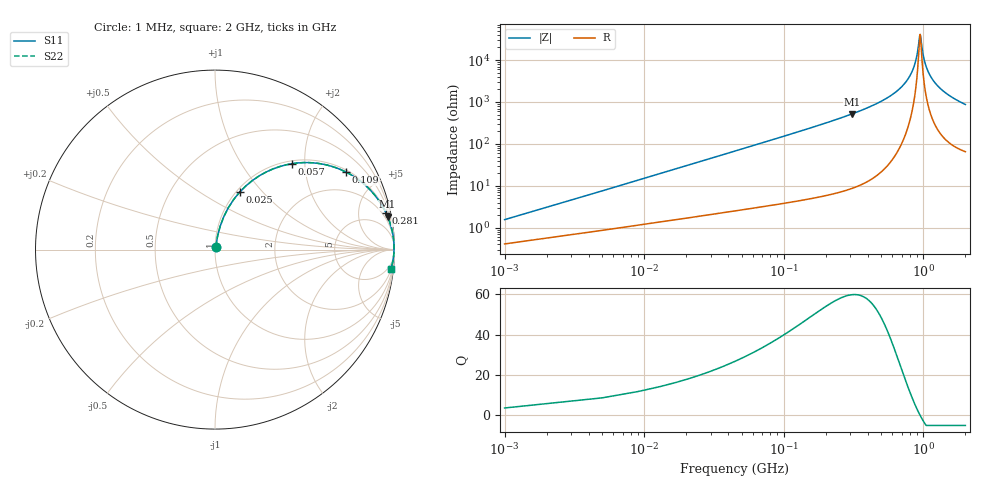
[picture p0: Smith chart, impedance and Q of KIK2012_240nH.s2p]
!version-2
!date-01.2022
!Series
# MHz S RI R 50
!Freq ReS11 ImS11 ReS21 ImS21 ReS12 ImS12 ReS22 ImS22
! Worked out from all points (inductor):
!   501 points, 1 MHz to 2 GHz, reference 50 ohm
!   read as one part in series: L = 240 nH near 9 MHz
!   highest Q = 59.8 at 309 MHz (marker M1), where L = 269 nH
!   self-resonance near 945 MHz
!   S11 on the Smith chart (normalised r, x): 1 MHz: 1.01, +0.03; 25 MHz: 1.04, +0.75; 57 MHz: 1.06, +1.73; 109 MHz: 1.08, +3.33; 281 MHz: 1.16, +9.29; 2 GHz: 2, -17
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1  0.00433 0.015  0.9957 -0.015  0.9957 -0.015  0.00433 0.015
13  0.0491 0.1839  0.9509 -0.1839  0.9509 -0.1839  0.0491 0.1839
25  0.1369 0.3196  0.8631 -0.3196  0.8631 -0.3196  0.1369 0.3196
37  0.2471 0.4113  0.7529 -0.4113  0.7529 -0.4113  0.2471 0.4113
57  0.4292 0.4787  0.5708 -0.4787  0.5708 -0.4787  0.4292 0.4787
109  0.7303 0.4319  0.2697 -0.4319  0.2697 -0.4319  0.7303 0.4319
173  0.8745 0.3216  0.1255 -0.3216  0.1255 -0.3216  0.8745 0.3216
281  0.9526 0.2042  0.0474 -0.2042  0.0474 -0.2042  0.9526 0.2042
309  0.9617 0.1838  0.0383 -0.1838  0.0383 -0.1838  0.9617 0.1838
337  0.9687 0.166  0.0313 -0.166  0.0313 -0.166  0.9687 0.166
669  0.9957 0.0494  0.00432 -0.0494  0.00432 -0.0494  0.9957 0.0494
773  0.9972 0.0286  0.00282 -0.0286  0.00282 -0.0286  0.9972 0.0286
849  0.9976 0.0153  0.0024 -0.0153  0.0024 -0.0153  0.9976 0.0153
897  0.9977 0.00766  0.00234 -0.00766  0.00234 -0.00766  0.9977 0.00766
945  0.9976 0.000398  0.00242 -0.000398  0.00242 -0.000398  0.9976 0.000398
957  0.9975 -0.00136  0.00246 0.00136  0.00246 0.00136  0.9975 -0.00136
1001  0.9973 -0.00761  0.00266 0.00761  0.00266 0.00761  0.9973 -0.00761
1049  0.997 -0.0141  0.00297 0.0141  0.00297 0.0141  0.997 -0.0141
1117  0.9964 -0.0229  0.00357 0.0229  0.00357 0.0229  0.9964 -0.0229
1337  0.9936 -0.0485  0.00643 0.0485  0.00643 0.0485  0.9936 -0.0485
1669  0.9872 -0.0817  0.0128 0.0817  0.0128 0.0817  0.9872 -0.0817
2000  0.979 -0.1108  0.021 0.1108  0.021 0.1108  0.979 -0.1108
